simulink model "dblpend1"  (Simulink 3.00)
settings: Solver=ode45  SolverMode=SingleTasking  StartTime=0  StopTime=10000  MaxStep=0.05  RelTol=1e-5  AbsTol=1e-6
PreLoadFcn:
  | l21=5;w21=5;n1=1/4;e1=1/2;

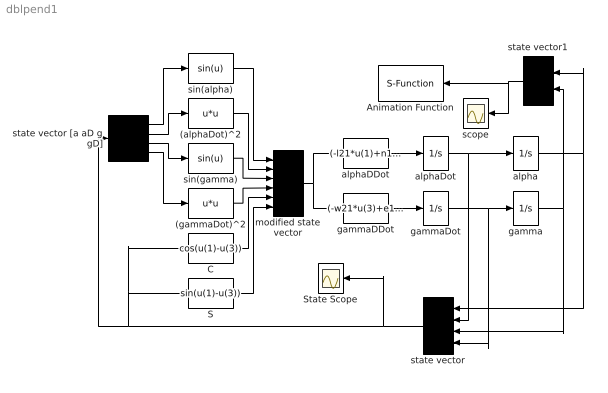
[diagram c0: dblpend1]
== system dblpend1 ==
  (alphaDot)^2 : Fcn  Expr=u*u
  (gammaDot)^2 : Fcn  Expr=u*u
  Animation Function : S-Function  Orientation=left  FunctionName=pndanim2  Parameters=0.05  PortCounts=[]  SFunctionModules=''
  C : Fcn  Expr=cos(u(1)-u(3))
  S : Fcn  Expr=sin(u(1)-u(3))
  State Scope : Scope
  alpha : Integrator  ExternalReset=none  InitialConditionSource=internal  InitialCondition=100*(pi/180)  LimitOutput=off  UpperSaturationLimit=inf  LowerSaturationLimit=-inf  ShowSaturationPort=off  ShowStatePort=off  AbsoluteTolerance=auto
  alphaDDot : Fcn  Expr=(-l21*u(1)+n1*w21*u(5)*u(3)-n1*e1*u(5)*u(6)*u(2)-n1*u(6)*u(4))/(1-n1*e1*u(5)*u(5))
  alphaDot : Integrator  ExternalReset=none  InitialConditionSource=internal  InitialCondition=0  LimitOutput=off  UpperSaturationLimit=inf  LowerSaturationLimit=-inf  ShowSaturationPort=off  ShowStatePort=off  AbsoluteTolerance=auto
  gamma : Integrator  ExternalReset=none  InitialConditionSource=internal  InitialCondition=0*(pi/180)  LimitOutput=off  UpperSaturationLimit=inf  LowerSaturationLimit=-inf  ShowSaturationPort=off  ShowStatePort=off  AbsoluteTolerance=auto
  gammaDDot : Fcn  Expr=(-w21*u(3)+e1*l21*u(5)*u(1)+n1*e1*u(5)*u(6)*u(4)+e1*u(6)*u(2))/(1-n1*e1*u(5)*u(5))
  gammaDot : Integrator  ExternalReset=none  InitialConditionSource=internal  InitialCondition=0  LimitOutput=off  UpperSaturationLimit=inf  LowerSaturationLimit=-inf  ShowSaturationPort=off  ShowStatePort=off  AbsoluteTolerance=auto
  modified state vector : Mux  Inputs=6
  scope : Scope
  sin(alpha) : Fcn  Expr=sin(u)
  sin(gamma) : Fcn  Expr=sin(u)
  state vector : Mux  Orientation=left  Inputs=4
  state vector [a aD g gD] : Demux  Outputs=4
  state vector1 : Mux  Orientation=left  Inputs=2
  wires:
  state vector1/1 -> Animation Function/1, scope/1
  alphaDDot/1 -> alphaDot/1
  gammaDDot/1 -> gammaDot/1
  alphaDot/1 -> alpha/1, state vector/2
  gammaDot/1 -> gamma/1, state vector/4
  alpha/1 -> state vector/1, state vector1/1
  gamma/1 -> state vector/3, state vector1/2
  state vector/1 -> state vector [a aD g gD]/1, C/1, S/1, State Scope/1
  S/1 -> modified state vector/6
  C/1 -> modified state vector/5
  (gammaDot)^2/1 -> modified state vector/4
  sin(gamma)/1 -> modified state vector/3
  (alphaDot)^2/1 -> modified state vector/2
  sin(alpha)/1 -> modified state vector/1
  state vector [a aD g gD]/4 -> (gammaDot)^2/1
  state vector [a aD g gD]/3 -> sin(gamma)/1
  state vector [a aD g gD]/2 -> (alphaDot)^2/1
  state vector [a aD g gD]/1 -> sin(alpha)/1
  modified state vector/1 -> alphaDDot/1, gammaDDot/1
